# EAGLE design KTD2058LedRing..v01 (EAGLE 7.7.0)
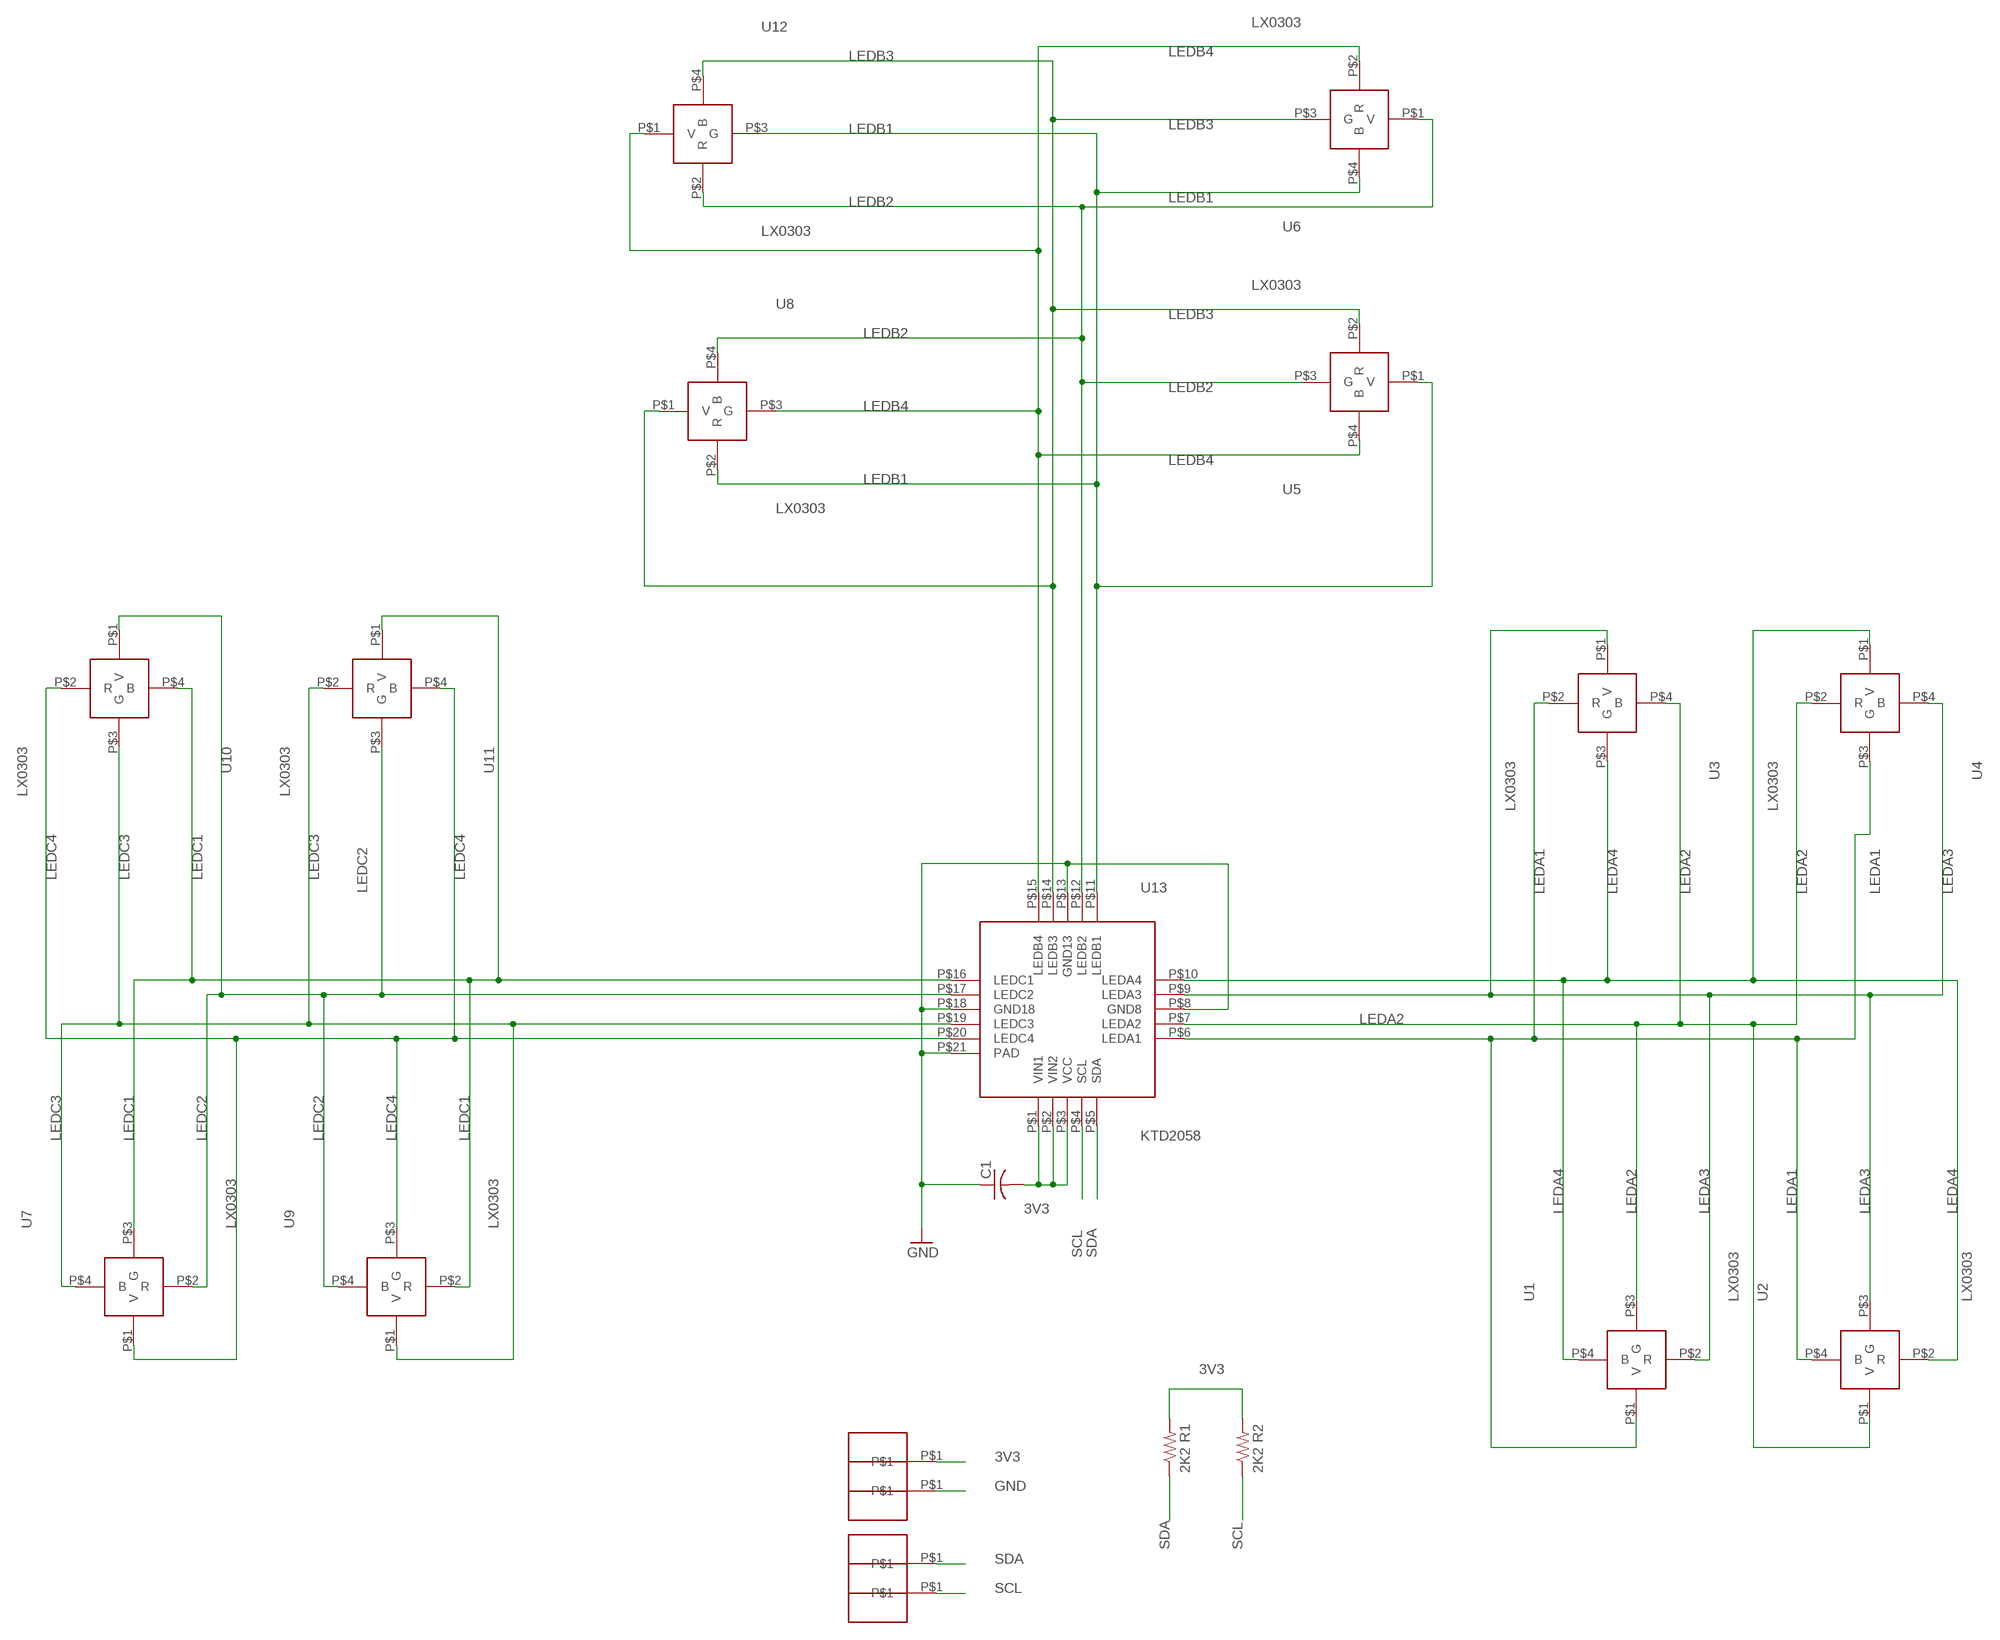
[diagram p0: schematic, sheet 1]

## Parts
C1  C-USC0603K  [C0603K]
R1  2K2  R-US_  [R0402_B]
R2  2K2  R-US_  [R0402_B]
U1  LX0303  [LX0303]
U2  LX0303  [LX0303]
U3  LX0303  [LX0303]
U4  LX0303  [LX0303]
U5  LX0303  [LX0303]
U6  LX0303  [LX0303]
U7  LX0303  [LX0303]
U8  LX0303  [LX0303]
U9  LX0303  [LX0303]
U10  LX0303  [LX0303]
U11  LX0303  [LX0303]
U12  LX0303  [LX0303]
U13  KTD2058  [KTD2058]
U$1  HN01  [HN01]
U$2  HN01  [HN01]
U$3  HN01  [HN01]
U$4  HN01  [HN01]

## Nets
3V3: C1.2 R1.2 R2.2 U13.P$1(VIN1) U13.P$2(VIN2) U13.P$3(VCC) U$4.P$1
GND: C1.1 U13.P$8(GND8) U13.P$13(GND13) U13.P$18(GND18) U13.P$21(PAD) U$3.P$1
LEDA1: U1.P$1(V) U2.P$4(B) U3.P$2(R) U4.P$3(G) U13.P$6(LEDA1)
LEDA2: U1.P$3(G) U2.P$1(V) U3.P$4(B) U4.P$2(R) U13.P$7(LEDA2)
LEDA3: U1.P$2(R) U2.P$3(G) U3.P$1(V) U4.P$4(B) U13.P$9(LEDA3)
LEDA4: U1.P$4(B) U2.P$2(R) U3.P$3(G) U4.P$1(V) U13.P$10(LEDA4)
LEDB1: U5.P$1(V) U6.P$4(B) U8.P$2(R) U12.P$3(G) U13.P$11(LEDB1)
LEDB2: U5.P$3(G) U6.P$1(V) U8.P$4(B) U12.P$2(R) U13.P$12(LEDB2)
LEDB3: U5.P$2(R) U6.P$3(G) U8.P$1(V) U12.P$4(B) U13.P$14(LEDB3)
LEDB4: U5.P$4(B) U6.P$2(R) U8.P$3(G) U12.P$1(V) U13.P$15(LEDB4)
LEDC1: U7.P$3(G) U9.P$2(R) U10.P$4(B) U11.P$1(V) U13.P$16(LEDC1)
LEDC2: U7.P$2(R) U9.P$4(B) U10.P$1(V) U11.P$3(G) U13.P$17(LEDC2)
LEDC3: U7.P$4(B) U9.P$1(V) U10.P$3(G) U11.P$2(R) U13.P$19(LEDC3)
LEDC4: U7.P$1(V) U9.P$3(G) U10.P$2(R) U11.P$4(B) U13.P$20(LEDC4)
SCL: R2.1 U13.P$4(SCL) U$1.P$1
SDA: R1.1 U13.P$5(SDA) U$2.P$1

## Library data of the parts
C1 = rcl:C-US: CAPACITOR, American symbol
R1 R2 = Spark:R-US_: 0402 Resistor
U1-U12 = Kris:LX0303: LX0303SUIP rgb led https://media.digikey.com/pdf/Data%20Sheets/Lumex%20PDFs/SML-LX0303SIUPGUSB_PA_10-26-17.pdf
U13 = Kris:KTD2058: KTD2058 36-channel rgb led driver
U$1-U$4 = PWSONN6:HN01

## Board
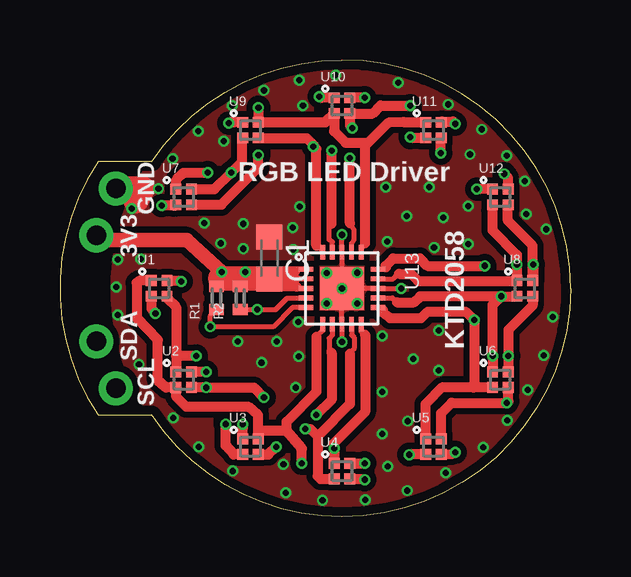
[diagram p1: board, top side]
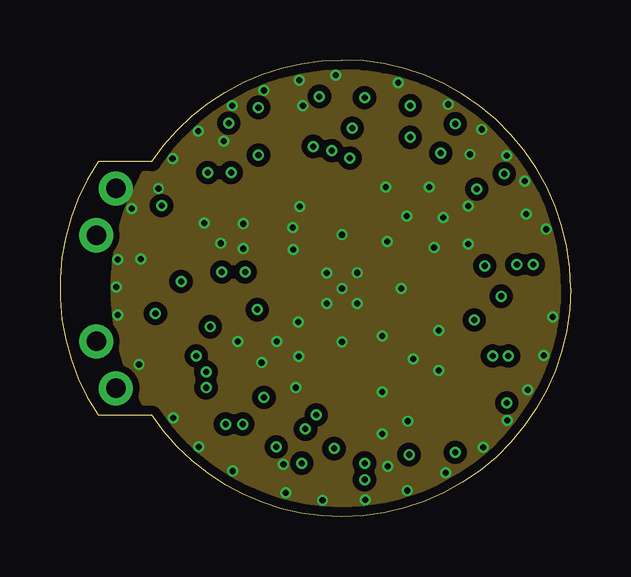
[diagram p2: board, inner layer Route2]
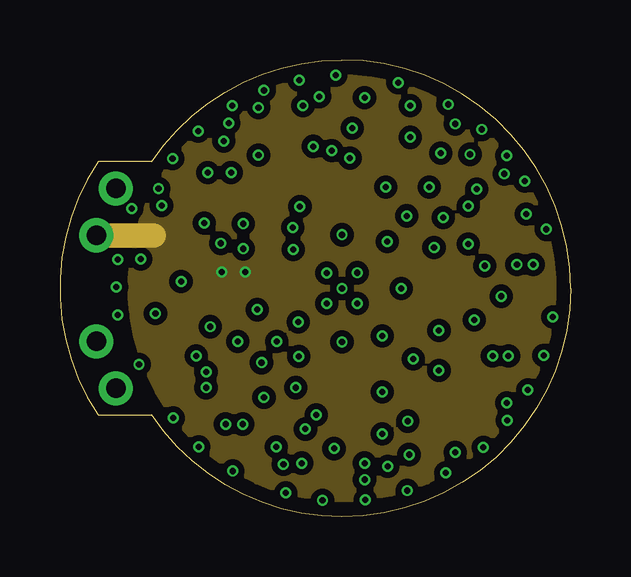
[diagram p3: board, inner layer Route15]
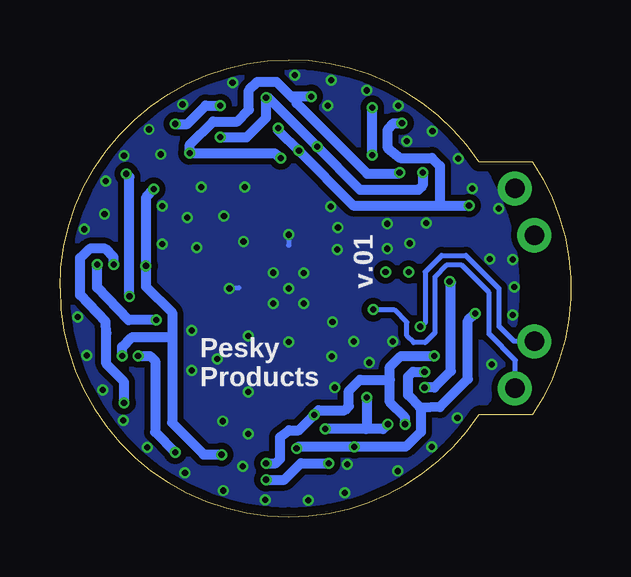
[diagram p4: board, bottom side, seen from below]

Size 21.27 x 19.05 mm. Coordinates in mm from the lower left corner, seen from the top.
Outline: 3.82,14.81 1.59,14.81 arc67 1.59,4.24 3.82,4.24 arc56 11.75,0 arc90 21.27,9.52 arc90 11.75,19.05 arc56 3.82,14.81
Copper layers (1*2*15*16): Top 0.035559375mm / dielectric 0.17018125mm / Route2 0.01778125mm / dielectric 47mil / Route15 0.01778125mm / dielectric 0.17018125mm / Bottom 0.035559375mm
Design rules "OSHPark-4layer *": minimum track width 5mil, minimum drill 10mil, track to track 5mil, track to pad 5mil, pad to pad 5mil, via to via 5mil, smd to smd 5mil, copper to edge 15mil, drill to drill 6mil, minimum pad ring 4mil, minimum via ring 4mil, stop-mask expansion 4mil, vias tented up to drill 20mil, thermal gap 10mil

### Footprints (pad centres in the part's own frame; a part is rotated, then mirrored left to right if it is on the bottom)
C0603K = smd 1.05 x 1.08: 1 -0.875,0; 2 0.875,0
R0402_B = smd 0.457 x 0.61: 1 -0.483,0; 2 0.483,0
LX0303 = smd 0.45 x 0.45: P$1 -0.325,0.325; P$2 0.325,0.325; P$3 0.325,-0.325; P$4 -0.325,-0.325
KTD2058 = smd 0.2 x 0.6: P$1 -0.8,-1.5; P$2 -0.4,-1.5; P$3 0,-1.5; P$4 0.4,-1.5; P$5 0.8,-1.5; P$11 0.8,1.5; P$12 0.4,1.5; P$13 0,1.5; P$14 -0.4,1.5; P$15 -0.8,1.5 | smd 0.6 x 0.2: P$6 1.5,-0.8; P$7 1.5,-0.4; P$8 1.5,0; P$9 1.5,0.4; P$10 1.5,0.8; P$16 -1.5,0.8; P$17 -1.5,0.4; P$18 -1.5,0; P$19 -1.5,-0.4; P$20 -1.5,-0.8 | smd 1.8 x 1.8: P$21 0,0
HN01 = drill 0.813 pad 1.422: P$1 0,0

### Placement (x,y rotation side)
C1  8.73,10.8 270 top
R1  6.52,9.12 90 top
R2  7.51,9.12 90 top
U1  4.13,9.52 0 top
U2  5.15,5.72 0 top
U3  7.94,2.93 0 top
U4  11.75,1.91 0 top
U5  15.56,2.93 0 top
U6  18.35,5.72 0 top
U7  5.15,13.34 0 top
U8  19.37,9.52 0 top
U9  7.94,16.12 0 top
U10  11.75,17.14 0 top
U11  15.56,16.12 0 top
U12  18.35,13.34 0 top
U13  11.75,9.52 270 top
U$1  2.33,5.36 0 top
U$2  1.51,7.32 0 top
U$3  2.33,13.69 0 top
U$4  1.51,11.73 0 top

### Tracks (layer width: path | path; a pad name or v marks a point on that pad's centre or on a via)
3V3  (via drill 0.25)
  Top 0.203: 8.65,10.32 C1.2 | 8.54,9.93 C1.2 | 8.84,9.52 C1.2 | U13.P$1 9.81,10.32 9.79,10.24 | U13.P$2 9.83,9.93 9.82,9.93 | U13.P$3 9.92,9.52 9.84,9.6 | 6.67,9.93 R1.2 6.85,9.93 v6.75,10.21 | R2.2 7.38,9.91 7.36,9.93
  Top 0.406: 9.79,10.24 8.79,10.24 C1.2 | 9.82,9.93 8.41,9.93 C1.2 | 9.84,9.6 8.79,9.6 C1.2
  Top 0.61: 8.39,9.93 C1.2 | v6.75,10.21 5.27,11.53 1.72,11.53 U$4.P$1
  Top 1.016: 6.67,9.93 6.85,9.93 7.36,9.93 8.39,9.93
  Route15 1.016: 3.9,11.73 1.61,11.73 1.59,11.76
  other vias: 7.71,10.21
  pour Route15 (isolate 0.254, no thermals): 5.52,15.75 arc-90 17.98,15.75 arc-90 17.98,3.3 arc-90 5.52,3.3 arc-90
GND  (via drill 0.25)
  Top 0.203: v11.75,7.29 U13.P$8 11.75,9.5 11.72,9.52 | v11.75,11.76 U13.P$18 11.75,9.55 11.77,9.52 U13.P$13 v14.21,9.52
  Top 1.016: U$3.P$1 3.44,13.69 3.16,13.16
  Bottom 0.203: v11.75,11.76 11.75,11.33 11.72,11.33 | v14.21,9.52 13.81,9.55
  other vias: 11.75,9.52 12.38,10.18 11.11,10.16 11.11,8.89 12.38,8.89 7.64,11.18 7.18,17.14 13.63,11.48 11.5,18.41 14.09,18.11 14.72,6.58 9.95,6.68 4.71,4.11 8.5,17.78 10.12,17.14 4.69,14.94 5.76,16.08 6.82,15.67 10,12.93 9.72,11.15 7.64,12.22 6.01,12.24 2.4,10.72 3.29,6.35 7.41,7.32 5.78,2.92 9.82,5.38 8.4,6.43 9.03,7.32 7.2,1.91 9.41,0.99 9.31,2.18 12.72,0.71 14.47,1.09 16.07,1.83 13.65,2.11 14.49,3.99 13.43,5.21 13.43,7.54 15.79,7.77 15.79,6.1 13.43,3.45 17.64,2.9 18.63,4.01 19.5,5.28 20.54,8.33 20.16,6.73 20.26,11.99 19.37,14 19.42,12.62 17.01,11.38 17.01,12.95 15.59,11.23 13.58,13.74 15.38,13.74 15.97,12.47 14.44,12.55 18.61,15.06 17.57,16.15 16.17,17.2 17.08,15.11 9.97,18.21 4.1,13.69 2.99,12.85 9.69,12.07 6.7,11.4 9.92,8.13 2.4,8.41 3.37,10.74 10.94,0.69 2.35,9.58
  pour Bottom (isolate 0.254, no thermals): 5.01,16.26 arc-90 18.49,16.26 arc-90 18.49,2.79 arc-90 5.01,2.79 arc-90
  pour Route2 (isolate 0.254, no thermals): 5.01,16.26 arc-90 18.49,16.26 arc-90 18.49,2.79 arc-90 5.01,2.79 arc-90
  pour Top (isolate 0.254, no thermals): 5.01,16.26 arc-90 18.59,16.26 arc-90 18.59,2.79 arc-90 5.01,2.79 arc-90
LEDA1  (via drill 0.25)
  Top 0.203: U13.P$6 10.95,7.76 10.68,7.52
  Top 0.406: U1.P$1 3.31,9.85 3.19,9.75 3.19,8.28 4.08,7.37 4.08,5.69 4.41,5.39 U2.P$4 4.83,5.02 5.25,4.6 7.84,4.6 8.24,4.24 8.24,3.27 U3.P$2 8.26,3.58 9.44,3.58 | 10.68,7.52 10.68,5.21 9.44,3.96 9.44,3.58 | v10.07,2.24 10.07,2.84 9.44,3.58 | U4.P$3 12.58,1.58 v12.69,1.55
  Bottom 0.406: v12.69,1.55 11.93,1.55 11.24,2.24 v10.07,2.24
LEDA2  (via drill 0.25)
  Top 0.203: U13.P$7 11.35,7.58 11.22,7.44 11.22,6.93 11.32,6.83
  Top 0.406: U1.P$3 4.45,9.12 4.84,8.74 4.84,6.71 | 4.84,6.71 4.84,6.2 U2.P$1 | v5.68,6.71 4.84,6.71 | U4.P$2 12.66,2.23 v12.69,2.24 | 11.32,6.83 11.32,4.88 v10.68,4.24 | U3.P$4 7.24,2.6 6.9,2.97 v6.9,3.86
  Bottom 0.406: v6.9,3.86 6.9,4.14 7.53,4.78 7.53,5.72 | v5.68,6.71 7.08,6.71 7.53,6.25 7.53,5.72 | 7.53,5.72 8.78,5.72 9.23,5.26 9.23,4.62 9.41,4.45 10.5,4.45 10.66,4.29 v10.68,4.24 11.32,3.61 11.72,3.61 12.11,3.33 12.11,2.41 12.28,2.24 v12.69,2.24
LEDA3  (via drill 0.25)
  Top 0.203: U13.P$9 12.15,7.58 12.26,7.47 12.26,7.01 12.08,6.81
  Top 0.406: U1.P$2 4.95,9.85 v5.04,9.8 | U2.P$3 v6.09,5.39 8.09,5.39 v8.5,4.98 | 12.08,6.81 12.08,4.7 10.73,3.35 | 10.73,3.35 10.73,1.7 10.86,1.58 U4.P$4 | U3.P$1 7.61,3.71 v7.61,3.86 | v10.23,3.66 10.43,3.66 10.73,3.35
  Bottom 0.406: v6.09,5.39 6.05,5.39 5.68,5.39 4.99,6.08 4.99,9.75 v5.04,9.8 | 8.52,3.66 7.81,3.66 v7.61,3.86 | 8.52,3.66 v10.23,3.66 | v8.5,4.98 8.5,3.68 8.52,3.66
LEDA4  (via drill 0.25)
  Top 0.203: U13.P$10 12.55,7.71 12.71,7.59
  Top 0.406: U1.P$4 3.8,8.68 v3.98,8.48 | v6.09,6.05 U2.P$2 | 12.71,7.59 12.71,4.37 11.42,3.07 v11.42,2.84 U4.P$1 | U3.P$3 8.69,2.6 v9.01,2.92
  Bottom 0.406: v6.09,6.05 6.57,6.05 6.77,5.84 6.77,5.08 6.24,4.55 | v3.98,8.48 4.28,8.18 4.28,5.74 5.45,4.57 6.24,4.55 | v11.42,2.84 11.34,2.92 v9.01,2.92 6.87,2.92 6.24,3.53 6.24,4.52 6.29,4.57 6.24,4.55
LEDB1  (via drill 0.25)
  Top 0.203: U13.P$11 13.44,8.73 13.45,8.61
  Top 0.406: 13.45,8.61 13.45,8.51 13.76,8.28 15.05,8.28 15.33,8.56 16.91,8.56 v17.26,8.2 17.26,5.41 17.24,5.39 | U6.P$4 17.24,5.39 | U5.P$1 15.23,4.7 15.92,5.39 17.24,5.39 | U12.P$3 18.66,13 18.66,12.34 19.69,11.31 U8.P$2 19.73,9.88 v19.73,10.52
  Bottom 0.406: v17.26,8.2 18.43,8.2 19.73,9.55 v19.73,10.52
LEDB2  (via drill 0.25)
  Top 0.203: U13.P$12 13.85,9.12 14.04,8.94
  Top 0.406: U6.P$1 v18.02,6.71 18.02,8.84 v18.38,9.2 | U6.P$1 | 14.04,8.94 14.75,8.94 15,9.2 v18.38,9.2 | U12.P$2 18.67,14.14 v18.51,14.3 | v18.38,9.2 U8.P$4 | U5.P$3 16.36,2.63 v16.47,2.69
  Bottom 0.406: v18.38,9.2 18.38,14.17 v18.51,14.3 | v16.47,2.69 17.31,3.53 17.31,6.5 17.52,6.71 v18.02,6.71
LEDB3  (via drill 0.25)
  Top 0.203: U13.P$14 13.88,9.93 14.06,10.11 14.2,10.11 14.13,10.13
  Top 0.406: U12.P$4 | U5.P$2 15.88,4.31 16.32,4.75 v18.61,4.75 18.68,4.83 18.68,5.38 U6.P$3 | 19.04,10.92 U8.P$1 19.02,9.83 14.92,9.83 14.63,10.13 14.13,10.13 | 19.04,10.92 18.02,11.94 U12.P$4 | U12.P$4 | v19.04,10.52 19.04,10.92
  Bottom 0.406: v19.04,10.52 19.04,10.82 19.39,11.18 20.03,11.18 20.44,10.8 20.44,9.25 19.37,8.13 19.34,7.65 19.34,6.38 18.61,5.61 v18.61,4.75
LEDB4  (via drill 0.25)
  Top 0.203: U13.P$15 13.49,10.32 13.58,10.41
  Top 0.406: 13.58,10.41 13.55,10.46 13.58,10.46 13.88,10.77 15,10.77 15.31,10.46 v17.69,10.46 | U12.P$1 17.42,13.66 v17.36,13.66 | U5.P$4 14.55,2.6 v14.54,2.59 | U6.P$2 18.68,6.05 v18.68,6.71 18.68,7.8 19.69,8.81 U8.P$3
  Bottom 0.406: v17.36,13.66 17.69,13.31 v17.69,10.46 17.69,9.6 16.6,8.51 16.6,7.47 | 16.6,7.47 18.3,7.47 18.68,7.09 v18.68,6.71 | 16.6,7.47 16.6,3.92 15.29,2.6 14.55,2.6 v14.54,2.59
LEDC1  (via drill 0.25)
  Top 0.203: U13.P$16 12.55,11.16 12.71,11.41
  Top 0.406: 12.71,11.41 12.71,15.54 | U11.P$1 14.31,16.46 13.68,16.43 12.77,15.52 12.71,15.54 | U7.P$3 6.73,13.01 8.27,14.55 v8.27,15.09 | v8.27,17.07 U9.P$2 11.05,16.45 U10.P$4 11.42,16.07 11.9,15.6 12.71,15.6 12.71,15.54
  Bottom 0.406: v8.27,15.09 v8.27,17.07
LEDC2  (via drill 0.25)
  Top 0.203: U13.P$17 12.15,11.4 12.26,11.56 12.26,11.96 12.08,12.24
  Top 0.406: 12.08,12.24 v12.08,14.96 | v15.86,15.16 15.86,15.78 U11.P$3 | 11.44,17.49 U10.P$1 10.89,17.47 v10.81,17.53 | U7.P$2 6.44,13.66 v7.13,14.35 7.58,14.81 7.58,15.77 U9.P$4
  Bottom 0.406: v7.13,14.35 7.18,14.3 8.47,14.3 11.42,17.25 U10.P$1 11.59,17.47 11.65,17.53 | v12.08,14.96 12.33,15.16 v15.86,15.16 15.86,15.52 14.9,16.48 13.88,16.48 13.4,16.97 13.4,17.78 13.04,18.14 12.26,18.14 11.65,17.53 | v10.81,17.53 11.65,17.53
LEDC3  (via drill 0.25)
  Top 0.203: U13.P$19 11.35,11.47 11.22,11.56 11.22,12.14 11.32,12.22
  Top 0.406: 11.32,12.22 v11.32,15.27 | U10.P$3 | U10.P$3 13.02,16.82 13.35,17.14 v14.59,17.14 | U11.P$2 15.92,16.48 16.38,16.48 v16.47,16.38 | v4.23,12.98 4.72,12.97 4.79,12.97 U7.P$4 | U10.P$3 12.07,16.31 v12.18,16.2 | U9.P$1 7.24,16.45 7.13,16.46 v7.03,16.41
  Bottom 0.406: 5.4,12.98 9.06,12.98 v11.32,15.27 12.18,16.1 v12.18,16.2 | 5.4,12.98 v4.23,12.98 | 5.4,12.98 5.45,13.03 5.45,14.63 5.78,14.96 7.1,14.96 7.61,15.37 7.61,16.15 7.38,16.41 v7.03,16.41 | v16.47,16.38 15.97,16.38 15.2,17.14 v14.59,17.14
LEDC4  (via drill 0.25)
  Top 0.203: U13.P$20 10.95,11.06 10.68,11.3
  Top 0.406: 10.68,11.3 10.68,15.34 10.61,15.45 | U9.P$3 8.29,15.77 10.3,15.77 10.61,15.45 | U11.P$4 14.62,15.8 v14.59,15.82 | v12.69,17.47 12.18,17.47 U10.P$2 | U7.P$1 4.85,13.66 4.85,14.05 5.15,14.35 v6.16,14.35 | v10.56,15.44 10.61,15.44 10.61,15.45
  Bottom 0.406: v14.59,15.82 13.5,15.82 12.69,16.64 v12.69,17.47 12.59,17.47 v10.56,15.44 8.78,13.64 6.34,13.64 6.16,13.82 v6.16,14.35
SCL  (via drill 0.25)
  Top 0.203: R2.1 v8.22,8.64 8.98,8.64 9.46,9.12 U13.P$4
  Bottom 0.203: U$1.P$1 2.3,6.53 3.39,7.62 3.39,9.35 4.54,10.49 5.17,10.49 5.65,10.01 5.65,7.67 6.06,7.26 6.54,7.26 6.82,7.54 6.82,8.1 7.36,8.64 v8.22,8.64
SDA  (via drill 0.25)
  Top 0.203: U13.P$5 9.68,8.73 8.88,7.92 v6.26,7.92 6.26,8.38 R1.1
  Bottom 0.203: U$2.P$1 2.35,7.32 2.99,7.95 2.99,9.52 4.36,10.9 5.37,10.9 6.06,10.21 6.06,8.08 v6.26,7.92

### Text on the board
tPlace: RGB LED Driver | GND | 3V3 | SDA | KTD2058 | SCL
bPlace: v.01 | Pesky / Products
